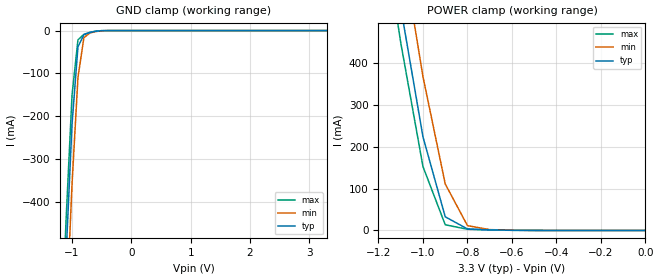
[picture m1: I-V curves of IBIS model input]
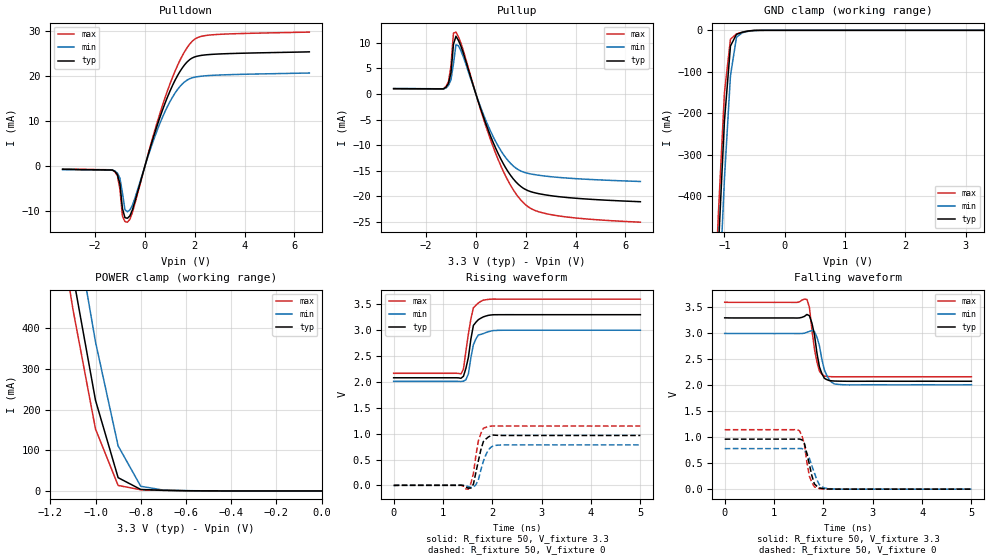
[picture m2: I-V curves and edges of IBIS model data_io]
| TSOP package &   Commercial  Operation
[IBIS Ver]   3.2
[Comment Char]   |_char
[File name]   as7c31024b_tsopc.ibs
[File Rev]   1.0
[Date]   May 19, 2004 4:10:13 PM
[Source]
Alliance Semiconductor Corporation
[Notes]
This model  is for TSOP package &
 Commercial  Operation
[Disclaimer]
Data is for modeling purpose only and is not guaranted.
This IBIS model is provided on an "AS IS" basis and Alliance Semiconductor makes
absolutely no warranty with respect to the information contained
herein.The entire risk as to quality and performance
is with the Customer. ACCORDINGLY, IN NO EVENT SHALL THE COMPANY BE
LIABLE FOR ANY DAMAGES, WHETHER IN CONTRACT OR TORT,INCLUDING ANY
LOST PROFITS OR OTHER INCIDENTAL, CONSEQUENTIAL, EXEMPLARY, OR
PUNITIVE DAMAGES ARISING OUT OF THE USE OR APPLICATION OF THE IBIS
model provided in this package.
[Copyright]
Alliance Semiconductor Corporation
| tsop Package & Commercial Operation.
[Component]   AS7C31024B_TSOPC
Si_location Pin
Timing_location Pin
[Manufacturer]   Alliance Semiconductor Corporation
[Package]
R_pkg   226.75m   113.8m   339.7m
L_pkg   5.159nH   3.003nH   7.315nH
C_pkg   0.7210pF   0.51pF   0.932pF
[Pin] signal_name   model_name
1   A11   input
2   A9   input
3   A8   input
4   A13   input
5   NWE   input
6   CE2   input
7   A15   input
8   VCC   input
9   NC   NC
10   A16   input
11   A14   input
12   A12   input
13   A7   input
14   A6   input
15   A5   input
16   A4   input
17   A3   input
18   A2   input
19   A1   input
20   A0   input
21   IO0   data_io
22   IO1   data_io
23   IO2   data_io
24   GND   GND
25   IO3   data_io
26   IO4   data_io
27   IO5   data_io
28   IO6   data_io
29   IO7   data_io
30   NCE1   input
31   A10   input
32   NOE   input
| Models and submodels in the file (2): input (Input), data_io (I/O)
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[Model]   input
Model_type Input
Vinh=2V
Vinl=0.8V
C_comp   4pF   4pF   4pF
[Model Spec]
[Temperature Range] 25   70   0
[Voltage Range]   3.3   3.0   3.6
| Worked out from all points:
|   GND clamp passes 1 mA (typ) near -0.56 V on its own axis
|   POWER clamp passes 1 mA (typ) near -0.65 V on its own axis
[GND Clamp]
-3.3V     -8.605A    -8.678A    -8.569A
-1.2V     -871.8mA   -1.032A    -786.6mA
-1.1V     -525.3mA   -681.9mA   -442.6mA
-1V       -219.6mA   -359.8mA   -151.4mA
-900mV    -38.16mA   -110mA     -21.74mA
-800mV    -9.652mA   -16.68mA   -8.786mA
-700mV    -4.621mA   -5.631mA   -4.129mA
-600mV    -1.581mA   -2.258mA   -1.211mA
-400mV    -22.59uA   -71.08uA   -10.05uA
3.3V      156pA      1.566uA    81.03pA
[POWER Clamp]
-3.3V     8.613A     8.687A     8.576A
-1.2V     879.9mA    1.042A     793.6mA
-1.1V     531.7mA    690.5mA    447.6mA
-1V       222.9mA    366.4mA    152.1mA
-900mV    32.63mA    110.9mA    13.56mA
-800mV    3.618mA    11.48mA    2.851mA
-700mV    1.463mA    2.037mA    1.288mA
0V        156pA      1.542nA    96.3pA
[Model]   data_io
Model_type I/O
Enable Active-High
Polarity Non-Inverting
Vinh=2V
Vinl=0.8V
Vref=1.728V
Vmeas=1.5V
Rref=168
Cref=30pF
C_comp   4pF   4pF   4pF
[Temperature Range] 25   70   0
[Voltage Range]   3.3   3.0   3.6
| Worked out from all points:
|   slope of the pulldown table from 0 to 0.495 V, typ, clamps not added: 54.6 ohm
|   slope of the pullup table from 0 to 0.495 V, typ, clamps not added: 70.3 ohm
|   GND clamp passes 1 mA (typ) near -0.56 V on its own axis
|   POWER clamp passes 1 mA (typ) near -0.65 V on its own axis
|   falling waveform, R_fixture 50, V_fixture 3.3: 20-80 % time 132ps typ, 153ps min, 130ps max; typ from 3.3 V to 2.08 V
|   falling waveform, R_fixture 50, V_fixture 0: 20-80 % time 145ps typ, 183ps min, 125ps max; typ from 0.964 V to 0.002 V
|   rising waveform, R_fixture 50, V_fixture 3.3: 20-80 % time 130ps typ, 130ps min, 144ps max; typ from 2.08 V to 3.3 V
|   rising waveform, R_fixture 50, V_fixture 0: 20-80 % time 140ps typ, 158ps min, 121ps max; typ from 0 V to 0.965 V
[Pullup]
-3.3V     1.05mA     1.087mA    1.024mA
-1.2V     1.343mA    1.17mA     1.474mA
-1.1V     2.093mA    1.672mA    2.412mA
-1V       4.162mA    2.808mA    5.487mA
-900mV    9.749mA    5.896mA    11.9mA
-800mV    11.31mA    9.656mA    12.11mA
-600mV    9.355mA    8.459mA    9.96mA
800mV     -10.66mA   -9.352mA   -11.68mA
1.4V      -15.96mA   -13.6mA    -17.92mA
1.9V      -18.41mA   -15.25mA   -21.23mA
3.1V      -19.94mA   -16.21mA   -23.66mA
6.6V      -21.06mA   -17.1mA    -25.06mA
[Pulldown]
-3.3V     -660uA     -727uA     -611uA
-1.2V     -1.16mA    -1.035mA   -1.221mA
-1V       -3.903mA   -2.651mA   -5.08mA
-900mV    -9.341mA   -5.846mA   -11.03mA
-800mV    -11.4mA    -9.637mA   -12.26mA
-700mV    -11.53mA   -10.09mA   -12.4mA
-500mV    -9.671mA   -8.648mA   -10.25mA
300mV     5.674mA    5.038mA    6.069mA
900mV     15.26mA    13.21mA    16.66mA
1.4V      20.98mA    17.67mA    23.43mA
1.9V      24.04mA    19.64mA    27.76mA
6.6V      25.41mA    20.71mA    29.8mA
[GND Clamp]
-3.3V     -8.605A    -8.678A    -8.569A
-1.2V     -871.7mA   -1.032A    -786.5mA
-1.1V     -525.2mA   -681.8mA   -442.5mA
-1V       -219.5mA   -359.7mA   -151.2mA
-900mV    -37.94mA   -109.8mA   -21.51mA
-800mV    -9.536mA   -16.55mA   -8.686mA
-700mV    -4.587mA   -5.581mA   -4.103mA
-600mV    -1.576mA   -2.248mA   -1.208mA
-400mV    -22.59uA   -71.06uA   -10.05uA
3.3V      156pA      1.566uA    81.03pA
[POWER Clamp]
-3.3V     8.613A     8.687A     8.576A
-1.2V     879.9mA    1.042A     793.6mA
-1.1V     531.7mA    690.5mA    447.6mA
-1V       222.9mA    366.4mA    152.1mA
-900mV    32.6mA     110.9mA    13.53mA
-800mV    3.604mA    11.47mA    2.839mA
-700mV    1.459mA    2.032mA    1.285mA
0V        156pA      1.542nA    96.3pA
[Falling Waveform]
R_fixture=50
V_fixture=3.3
V_fixture_min=3.0
V_fixture_max=3.6
0s        3.3V       3V         3.6V
1.667ns   3.365V     3.022V     3.654V
1.717ns   3.34V      3.039V     3.502V
1.768ns   3.198V     3.059V     3.071V
1.869ns   2.627V     2.931V     2.454V
1.919ns   2.357V     2.766V     2.275V
2.02ns    2.136V     2.296V     2.176V
2.121ns   2.092V     2.104V     2.169V
2.273ns   2.082V     2.022V     2.166V
5ns       2.079V     2.01V      2.166V
[Falling Waveform]
R_fixture=50
V_fixture=0
V_fixture_min=0
V_fixture_max=0
0s        963.8mV    781.9mV    1.146V
1.515ns   965.2mV    784.2mV    1.125V
1.566ns   952.3mV    782.5mV    1.032V
1.616ns   879.7mV    758.3mV    859.2mV
1.667ns   680.3mV    686.1mV    515mV
1.717ns   474.8mV    590.5mV    247.7mV
1.818ns   102.7mV    312.3mV    47.11mV
1.919ns   26.61mV    86.24mV    13.35mV
2.222ns   2.571mV    4.8mV      2.253mV
5ns       2.006mV    1.927mV    2.127mV
[Rising Waveform]
R_fixture=50
V_fixture=3.3
V_fixture_min=3.0
V_fixture_max=3.6
0s        2.079V     2.01V      2.165V
1.364ns   2.07V      2.007V     2.153V
1.414ns   2.108V     2.013V     2.244V
1.515ns   2.478V     2.156V     2.929V
1.566ns   2.831V     2.47V      3.218V
1.616ns   3.09V      2.719V     3.431V
1.717ns   3.202V     2.906V     3.524V
1.818ns   3.256V     2.933V     3.579V
2.172ns   3.298V     2.997V     3.598V
5ns       3.298V     2.998V     3.598V
[Rising Waveform]
R_fixture=50
V_fixture=0
V_fixture_min=0
V_fixture_max=0
0s        0V         0V         0V
1.364ns   4.258mV    3.891mV    1.324mV
1.515ns   -53.51mV   -22.05mV   -72.59mV
1.616ns   23.88mV    -36.41mV   228.7mV
1.717ns   474.8mV    109.6mV    860.2mV
1.818ns   846mV      465.1mV    1.104V
1.919ns   935.3mV    686.7mV    1.137V
2.02ns    972.8mV    767.4mV    1.149V
2.172ns   965.1mV    780.4mV    1.146V
5ns       964.6mV    782.9mV    1.146V
[Ramp]
R_load=50
dV/dt_r   5.788E-1/1.331E-10   4.697E-1/1.534E-10   6.878E-1/1.208E-10
dV/dt_f   7.324E-1/1.248E-10   5.938E-1/1.485E-10   8.605E-1/1.296E-10
|[End   data_io
